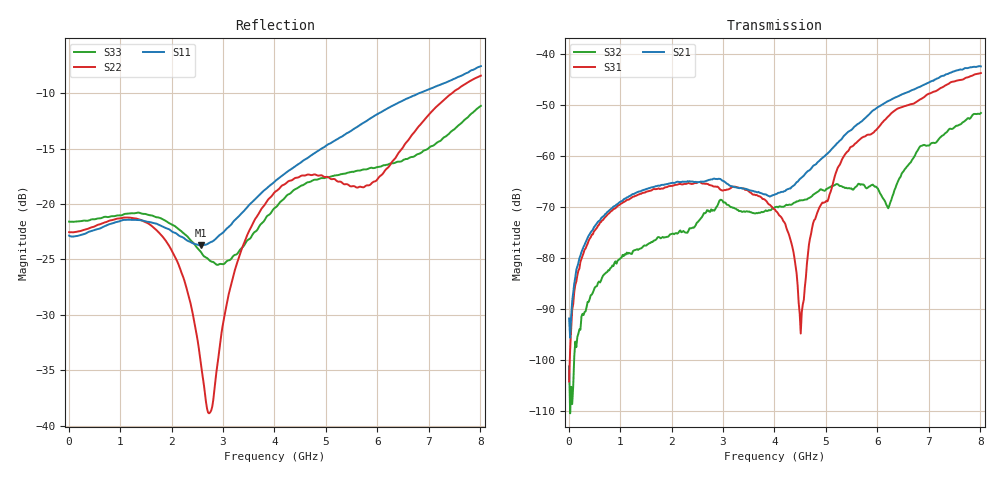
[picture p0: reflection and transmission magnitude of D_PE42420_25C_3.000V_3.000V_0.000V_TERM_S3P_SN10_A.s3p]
! Device ID: PE42420
! Serial: 10
! Insertion: A
! Temp: 25C
! VDD: 3.000
! Control_Hi: 3.000
! Control_Lo: 0.000
! Logic State: TERM
! Port 1: RFC
! Port 2: RF1
! Port 3: RF2
! V1 = 0.00
! V2 = 0.00
! V3 = 0.00
! IDD: 1.161621e-04
#  Hz  S  RI  R  50
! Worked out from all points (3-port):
!   401 points, 10 MHz to 8.01 GHz, reference 50 ohm
!   strongest paths, dB at 10 MHz, 2.01 GHz, 4.01 GHz, 6.01 GHz, 8.01 GHz:
!     S21: -91.9, -65.3, -67.6, -50.5, -42.5
!     S31: -104.3, -65.9, -70.6, -54.5, -43.8
!     S32: -101.3, -75.3, -70.1, -66.5, -51.6
!   lowest |S11| = -23.7 dB at 2.57 GHz (marker M1), VSWR 1.14, Z = 48.7 - j6.29 ohm
!   |S11| at or under -10 dB: start of sweep to 6.811 GHz
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1e7  0.0719 -0.00123  -3.41e-06 3.68e-06  -2.09e-06 -1.71e-05
     -3.5e-06 2.51e-05  0.0746 -0.000883  1.17e-05 -1.75e-05
     -6.12e-06 3.08e-08  -7.31e-06 4.53e-06  0.0832 -0.00103
1.73e9  0.0441 -0.0679  0.000222 0.000451  0.000291 0.000372
        0.000226 0.000454  0.0658 -0.0365  0.000108 0.000115
        0.000292 0.000373  0.000111 0.000113  0.0612 -0.0619
2.57e9  -0.00917 -0.0643  0.0003 0.000466  0.000467 0.000273
        0.000306 0.000467  0.0126 -0.0142  0.000214 0.000109
        0.000473 0.00027  0.00022 0.000108  0.0207 -0.0571
2.75e9  -0.0242 -0.0626  0.000318 0.000485  0.00047 0.000214
        0.000321 0.000485  -0.00358 -0.0109  0.000278 5.97e-05
        0.000468 0.000213  0.000275 6.3e-05  0.00695 -0.0549
4.01e9  -0.1226 -0.032  6.37e-05 0.000409  0.000298 -2.65e-06
        5.44e-05 0.000414  -0.1131 -0.00715  0.000246 -0.000171
        0.000296 -4.42e-06  0.000261 -0.000172  -0.0877 -0.0393
4.59e9  -0.1587 0.00114  -0.000271 0.000577  -5.18e-05 -6.43e-06
        -0.000294 0.000589  -0.1342 -0.00611  0.000238 -0.000265
        -5.11e-05 -8.25e-06  0.000256 -0.00027  -0.1197 -0.0284
5.49e9  -0.1956 0.0861  -0.00114 0.00128  -0.00114 0.000464
        -0.00118 0.00134  -0.114 0.0373  -0.000276 -0.00039
        -0.00114 0.00045  -0.000255 -0.000405  -0.1389 0.0106
6.21e9  -0.2019 0.1811  -0.00186 0.00276  -0.00214 0.00118
        -0.00187 0.00287  -0.0741 0.1261  -0.000324 4.03e-06
        -0.00213 0.00115  -0.000304 -2.87e-05  -0.1345 0.0682
6.83e9  -0.1775 0.2634  -0.00211 0.00412  -0.00283 0.00222
        -0.00207 0.00427  -0.0401 0.2239  -0.00123 2.41e-06
        -0.00283 0.00216  -0.00123 -3.07e-05  -0.1081 0.1301
8.01e9  -0.0421 0.4165  -0.000776 0.00726  -0.00353 0.0055
        -0.000603 0.00748  0.0202 0.3786  -0.00247 0.00091
        -0.00367 0.00531  -0.00248 0.000848  -0.00329 0.2772
